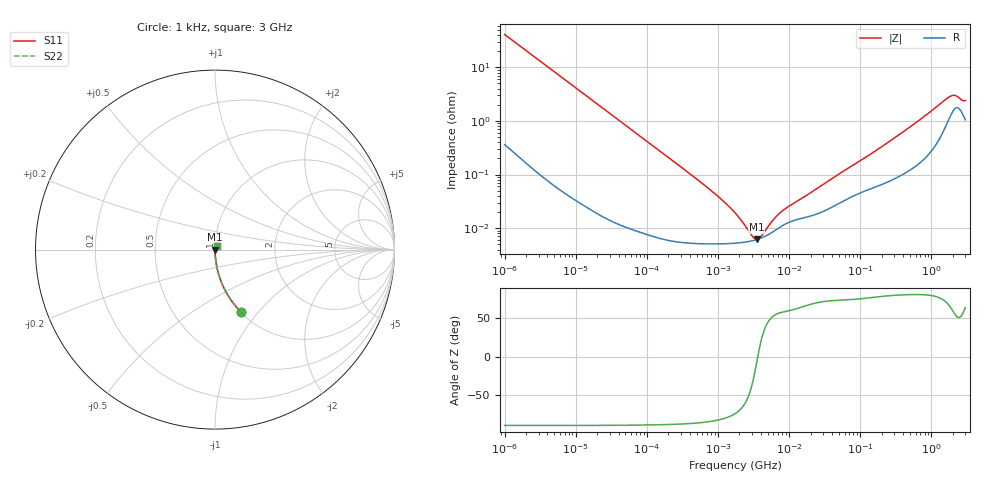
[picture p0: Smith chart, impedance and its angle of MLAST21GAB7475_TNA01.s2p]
! MLAST21GAB7475_TNA01  S-PARAMETER MODEL  ( Standard Model )
! Model Generated by TAIYO YUDEN Corporation (http://www.ty-top.com)
! Version 1.0
! TAIYO YUDEN Control No. 220601
! Copyright(c) 2010 TAIYO YUDEN CO.,LTD. All Rights Reserved.
! Product Description (link to TY-COMPAS)
! https://ds.yuden.co.jp/TYCOMPAS/or/detail?pn=MLAST21GAB7475KTNA01&u=M
! Products Name : Multilayer Ceramic Capacitors
! Characteristics :
!  Capacitance : 4.7 [uF] , Rated Voltage : 25 [V] , TCC : X7R
!  Case Size : 2.0 x 1.25 / 0.079 x 0.049 [mm/inch] , Thickness : 1.25 / 0.049 [mm/inch]
!  (Conditions: Temperature = 25 [degC] , DC Bias Voltage = 0 [V])
! External Node Assignments :
!  1  o---| |---o  2
! GND o---------o GND
! Frequency Range : 1kHz  -  3GHz  [ 401 STEP ]
# MHZ S RI R 50
! Freq[MHz].  S11 Real  S11 Imag  S21 Real  S21 Imag  S12 Real  S12 Imag  S22 Real  S22 Imag
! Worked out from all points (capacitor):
!   401 points, 1 kHz to 3 GHz, reference 50 ohm
!   read as one part in series: C = 3.87 uF near 1.077 kHz
!   lowest |Z| = 6.18 mohm at 3.517 MHz (marker M1)
!   series resonance near 3.617 MHz, so ESL is about 500 pH
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0.001  0.1461 -0.3488  0.8539 0.3488  0.8539 0.3488  0.1461 -0.3488
0.001685  0.0579 -0.2294  0.9421 0.2294  0.9421 0.2294  0.0579 -0.2294
0.003177  0.0175 -0.1274  0.9825 0.1274  0.9825 0.1274  0.0175 -0.1274
0.01216  0.00144 -0.034  0.9986 0.034  0.9986 0.034  0.00144 -0.034
0.147855  7.3e-05 -0.00283  0.9999 0.00283  0.9999 0.00283  7.3e-05 -0.00283
0.791611  5.11e-05 -0.000506  0.9999 0.000506  0.9999 0.000506  5.11e-05 -0.000506
1.238299  5.13e-05 -0.0003  0.9999 0.0003  0.9999 0.0003  5.13e-05 -0.0003
1.732051  5.24e-05 -0.000187  0.9999 0.000187  0.9999 0.000187  5.24e-05 -0.000187
2.514714  5.55e-05 -8.59e-05  0.9999 8.59e-05  0.9999 8.59e-05  5.55e-05 -8.59e-05
2.709407  5.64e-05 -6.77e-05  0.9999 6.77e-05  0.9999 6.77e-05  5.64e-05 -6.77e-05
3.517417  6.14e-05 -6.38e-06  0.9999 6.38e-06  0.9999 6.38e-06  6.14e-05 -6.38e-06
4.566395  7.04e-05 5.32e-05  0.9999 -5.32e-05  0.9999 -5.32e-05  7.04e-05 5.32e-05
4.919932  7.4e-05 7.02e-05  0.9999 -7.02e-05  0.9999 -7.02e-05  7.4e-05 7.02e-05
6.629817  9.42e-05 0.000137  0.9999 -0.000137  0.9999 -0.000137  9.42e-05 0.000137
8.291982  0.000114 0.000185  0.9999 -0.000185  0.9999 -0.000185  0.000114 0.000185
21.06097  0.000172 0.000447  0.9998 -0.000447  0.9998 -0.000447  0.000172 0.000447
256.0921  0.000765 0.00406  0.9992 -0.00406  0.9992 -0.00406  0.000765 0.00406
650.4536  0.00164 0.00981  0.9984 -0.00981  0.9984 -0.00981  0.00164 0.00981
1780.008  0.0117 0.0253  0.9883 -0.0253  0.9883 -0.0253  0.0117 0.0253
2144.796  0.0173 0.0237  0.9827 -0.0237  0.9827 -0.0237  0.0173 0.0237
2682.519  0.0144 0.0193  0.9856 -0.0193  0.9856 -0.0193  0.0144 0.0193
3000  0.0108 0.0211  0.9892 -0.0211  0.9892 -0.0211  0.0108 0.0211
